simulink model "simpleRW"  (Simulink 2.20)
settings: Solver=ode45  StartTime=min(t)  StopTime=max(t)  MaxStep=tick_interval  RelTol=1e-3  AbsTol=1e-6
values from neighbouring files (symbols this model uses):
  gain_in = 0    [run_simpleRW.m]
  N_ex = 300    [run_simpleRW.m]
  N_in = 150    [run_simpleRW.m]
  tick_interval = .001    (= 0.001)    [run_simpleRW.m]
undefined symbols (not defined in the file or in its folder): soundsc

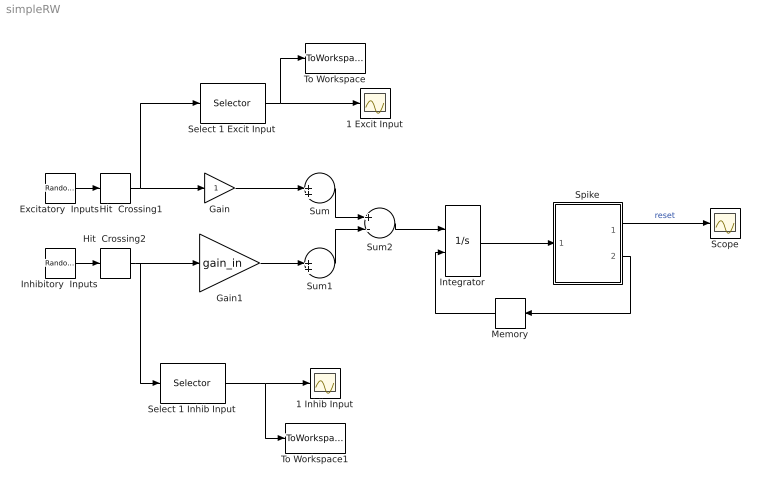
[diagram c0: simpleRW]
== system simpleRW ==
  1 Excit Input : Scope
  1 Inhib Input : Scope
  Excitatory  Inputs : RandomNumber  Mean=0  Variance=1  Seed=round(1000*rand(N_ex,1))  SampleTime=tick_interval
  Gain : Gain  Gain=1
  Gain1 : Gain  Gain=gain_in
  Hit  Crossing1 : HitCross  HitCrossingOffset=zval_ex  HitCrossingDirection=rising  ShowOutputPort=on
  Hit  Crossing2 : HitCross  HitCrossingOffset=zval_in  HitCrossingDirection=rising  ShowOutputPort=on
  Inhibitory  Inputs : RandomNumber  Mean=0  Variance=1  Seed=round(1000*rand(N_in,1))  SampleTime=tick_interval
  Integrator : Integrator  ExternalReset=rising  InitialConditionSource=internal  InitialCondition=0  LimitOutput=on  UpperSaturationLimit=inf  LowerSaturationLimit=0  ShowSaturationPort=off  ShowStatePort=off  AbsoluteTolerance=auto
  Memory : Memory  Orientation=left  X0=0  InheritSampleTime=off
  Scope : Scope
  Select 1 Excit Input : Selector  Elements=[1]  InputPortWidth=N_ex
  Select 1 Inhib Input : Selector  Elements=[1]  InputPortWidth=N_in
  Spike : Subsystem
  Sum : Sum  Inputs=1
  Sum1 : Sum  Inputs=1
  Sum2 : Sum  Inputs=+-
  To Workspace : ToWorkspace  VariableName=sin_ex  SampleTime=-1
  To Workspace1 : ToWorkspace  VariableName=sin_in  SampleTime=-1
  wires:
  Excitatory  Inputs/1 -> Hit  Crossing1/1
  Inhibitory  Inputs/1 -> Hit  Crossing2/1
  Select 1 Excit Input/1 -> 1 Excit Input/1, To Workspace/1
  Select 1 Inhib Input/1 -> To Workspace1/1, 1 Inhib Input/1
  Sum/1 -> Sum2/1
  Sum1/1 -> Sum2/2
  Sum2/1 -> Integrator/1
  Gain1/1 -> Sum1/1
  Hit  Crossing2/1 -> Select 1 Inhib Input/1, Gain1/1
  Gain/1 -> Sum/1
  Hit  Crossing1/1 -> Select 1 Excit Input/1, Gain/1
  Spike/1(Vm+spike) -> Scope/1  "reset"
  Spike/2(spike) -> Memory/1
  Memory/1 -> Integrator/2
  Integrator/1 -> Spike/1(Vm)

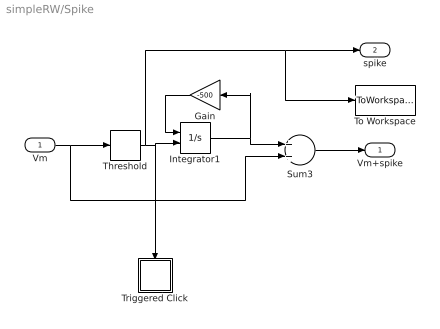
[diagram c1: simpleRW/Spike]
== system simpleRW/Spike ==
  Vm : Inport  Port=1  PortWidth=-1  SampleTime=-1
  Gain : Gain  Orientation=left  Gain=-500
  Integrator1 : Integrator  ExternalReset=rising  InitialConditionSource=internal  InitialCondition=1  LimitOutput=off  UpperSaturationLimit=inf  LowerSaturationLimit=-inf  ShowSaturationPort=off  ShowStatePort=off  AbsoluteTolerance=auto
  Sum3 : Sum  Inputs=++
  Threshold : HitCross  HitCrossingOffset=spike_threshold  HitCrossingDirection=rising  ShowOutputPort=on
  To Workspace : ToWorkspace  VariableName=sout  SampleTime=-1
  Triggered Click : Subsystem
  Vm+spike : Outport  Port=1  InitialOutput=0
  spike : Outport  Port=2  InitialOutput=0
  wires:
  Gain/1 -> Integrator1/1
  Sum3/1 -> Vm+spike/1
  Vm/1 -> Threshold/1, Sum3/2
  Threshold/1 -> spike/1, To Workspace/1, Integrator1/2, Triggered Click/Trigger
  Integrator1/1 -> Gain/1, Sum3/1

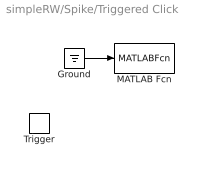
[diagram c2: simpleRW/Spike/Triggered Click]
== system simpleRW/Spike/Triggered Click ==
  Trigger : TriggerPort  TriggerType=rising
  Ground : Ground
  MATLAB Fcn : MATLABFcn  MATLABFcn=soundsc([0 0 1 1 1 0 0 0])  OutputWidth=0
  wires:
  Ground/1 -> MATLAB Fcn/1
